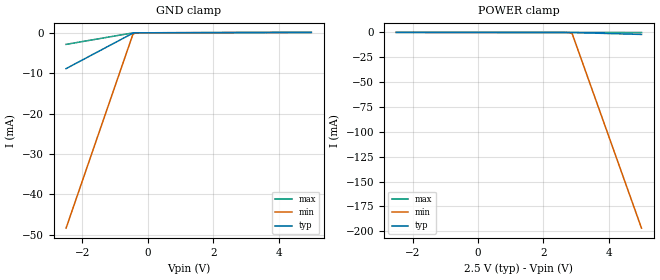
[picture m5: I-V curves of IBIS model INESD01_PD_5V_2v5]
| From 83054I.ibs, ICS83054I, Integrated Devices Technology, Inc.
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[Model] INESD01_PD_5V_2v5
Model_type   Input
Polarity   Non-Inverting
Vinl = 0.8V
Vinh = 2.0V
|   typ   min   max
C_comp   2pF   1.5pF   2.5pF
|   typ   min   max
[Voltage range]  2.5V   2.375V   2.625V
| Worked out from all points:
|   GND clamp passes 1 mA (typ) near -0.67 V on its own axis
[GND_clamp]
|Voltage   I(typ)   I(min)   I(max)
-2.5V     -8.873mA   -48.37mA   -2.87mA
-454.5mV  -90.52uA   -342uA     -24.79uA
-378.8mV  -21.06uA   -68.59uA   -9.129uA
-227.3mV  -4.664uA   -6.183uA   -4.627uA
5V        98.01uA    94.31uA    101.7uA
[POWER_clamp]
|Voltage   I(typ)   I(min)   I(max)
-2.5V     97.98uA    91.95uA    104.2uA
2.652V    -2.989uA   -11.36uA   -539.2nA
2.879V    -21.06uA   -1.086mA   -5.176uA
5V        -1.966mA   -196.9mA   -55.09uA
